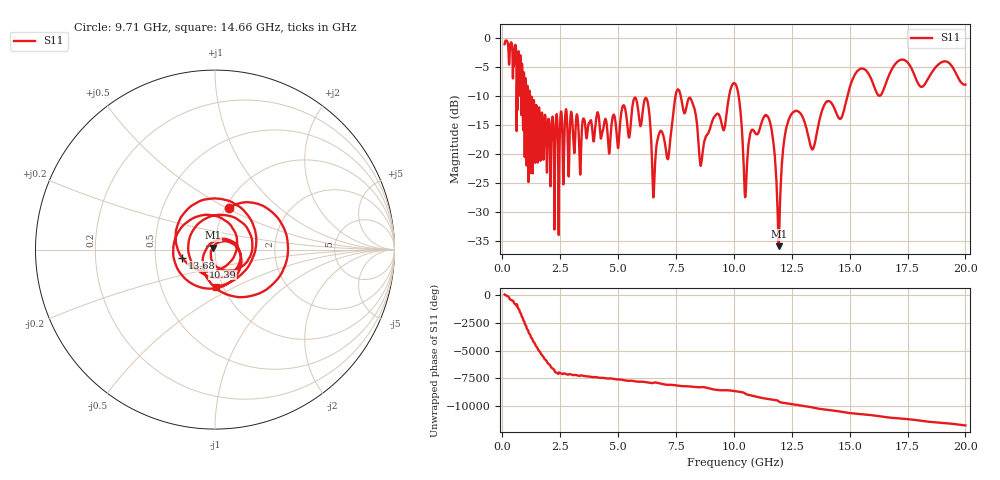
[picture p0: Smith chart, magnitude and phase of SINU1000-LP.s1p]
!Keysight Technologies,P9374A,MY57211922,A.15.40.13
!Date: Friday, July 10, 2026 13:44:15
!Correction: S11(C  1-Port  )
!S1P File: Measurement: S11:
# Hz S  dB  R 50
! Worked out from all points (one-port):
!   1991 points, 100 MHz to 20 GHz, reference 50 ohm
!   lowest |S11| = -36.0 dB at 11.94 GHz (marker M1), VSWR 1.03, Z = 48.8 + j0.985 ohm
!   |S11| at or under -10 dB: 1.184 GHz to 7.482 GHz (6.297 GHz wide, 145 % of centre); 7.706 GHz to 9.795 GHz (2.09 GHz wide, 23.9 % of centre); 10.21 GHz to 14.91 GHz (4.699 GHz wide, 37.4 % of centre)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
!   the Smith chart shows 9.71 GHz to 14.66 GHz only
!   S11 on the Smith chart (normalised r, x): 9.71 GHz: 1.05, +0.51; 10.39 GHz: 0.86, -0.16; 13.68 GHz: 0.69, -0.07; 14.66 GHz: 0.93, -0.40
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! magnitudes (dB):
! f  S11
! 100 MHz  -1.1
! 780 MHz  -3.0
! 1.13 GHz  -24.9
! 2.59 GHz  -15.8
! 5.08 GHz  -15.2
! 6.22 GHz  -10.4
! 6.55 GHz  -26.1
! 6.8 GHz  -16.3
! 7.18 GHz  -20.5
! 7.57 GHz  -8.9
! 8.23 GHz  -11.4
! 8.58 GHz  -22.0
! 9.71 GHz  -12.3
! 10.05 GHz  -7.9
! 10.39 GHz  -18.8
! 10.51 GHz  -26.9
! 10.74 GHz  -16.2
! 11.48 GHz  -13.6
! 11.7 GHz  -17.7
! 11.94 GHz  -36.0
! 12.19 GHz  -17.2
! 12.54 GHz  -12.9
! 13.38 GHz  -19.3
! 13.68 GHz  -14.5
! 14.66 GHz  -13.7
! 15.03 GHz  -8.2
! 17.52 GHz  -4.3
! 20 GHz  -8.1
